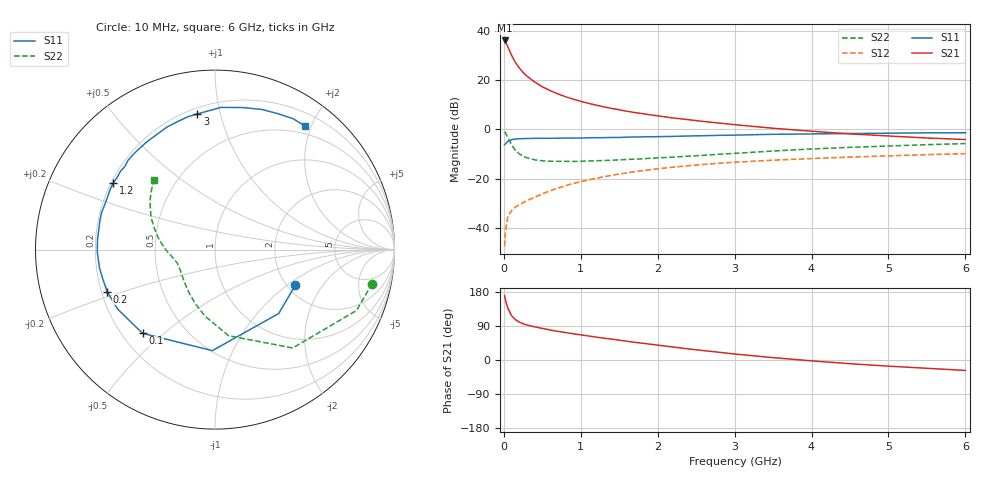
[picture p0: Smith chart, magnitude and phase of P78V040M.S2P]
! SIEMENS Small Signal Semiconductors
! BFP196
! Si NPN RF Bipolar Junction Transistor in SOT143
! VCE = 8 V  IC = 40 mA
! Common Emitter S-Parameters:  May  1996
# GHz  S  MA  R  50
!  f  S11  S21  S12  S22
! GHz  MAG  ANG  MAG  ANG  MAG  ANG  MAG  ANG
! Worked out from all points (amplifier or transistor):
!   36 points, 10 MHz to 6 GHz, reference 50 ohm
!   highest |S21| = 36.2 dB at 10 MHz (marker M1)
!   |S21| within 3 dB of that: start of sweep to 58.2 MHz
!   unconditionally stable (mu >= 1): 546.5 MHz to 4.494 GHz
!   at 250 MHz: K = 0.75, MSG = 26.5 dB, |S12| = -29.8 dB
!   at 1.4 GHz: K = 1.09, MAG = 11.8 dB, |S12| = -18.7 dB
!   at 6 GHz: K = 0.97, MSG = 2.9 dB, |S12| = -9.9 dB
!   S11 on the Smith chart (normalised r, x): 10 MHz: 2.22, -1.15; 100 MHz: 0.28, -0.43; 200 MHz: 0.22, -0.18; 1.2 GHz: 0.21, +0.29; 3 GHz: 0.24, +0.85; 6 GHz: 0.38, +1.91
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0.01  0.4898 -23.7  64.37 169.7  0.0042 79.7  0.8959 -12.2
0.02  0.5028 -45.1  60.9 159.5  0.0081 73.7  0.8581 -23.3
0.05  0.5632 -91.5  48.77 137.6  0.0164 57.4  0.6984 -51.7
0.1  0.6169 -130.9  32.24 117.0  0.0224 47.1  0.4859 -81.0
0.15  0.6358 -148.6  23.1 106.5  0.0263 45.9  0.3756 -98.4
0.2  0.6448 -158.7  17.86 100.1  0.0292 47.7  0.3186 -110.5
0.25  0.6467 -166.0  14.38 95.7  0.0322 48.8  0.283 -120.2
0.3  0.6514 -170.9  12.11 92.5  0.0354 50.9  0.2638 -127.0
0.4  0.6559 -178.8  9.188 87.5  0.0415 54.1  0.2405 -137.5
0.5  0.6571 175.3  7.354 83.3  0.0485 56.4  0.2293 -144.8
0.6  0.6567 170.5  6.146 79.3  0.0563 57.9  0.2248 -149.7
0.7  0.6615 165.5  5.289 75.5  0.0636 59.0  0.2235 -153.5
0.9  0.6631 157.8  4.116 69.4  0.0792 58.3  0.2225 -159.2
1.1  0.6732 150.4  3.384 63.4  0.0935 57.5  0.2272 -163.0
1.2  0.678 146.7  3.107 60.4  0.1011 56.7  0.2297 -164.7
1.7  0.6991 130.7  2.197 46.7  0.1374 51.0  0.2474 -172.5
2.2  0.7185 116.9  1.706 34.3  0.1699 44.3  0.2722 -179.3
3  0.7624 97.4  1.246 15.8  0.2147 32.9  0.325 167.7
3.5  0.793 87.6  1.053 6.2  0.2358 26.3  0.3621 159.9
4.5  0.8236 71.4  0.81 -9.8  0.2724 14.7  0.4302 147.0
5.5  0.8493 59.2  0.667 -21.9  0.3053 4.2  0.4878 136.4
6  0.8515 53.7  0.621 -27.6  0.3201 -1.5  0.5137 131.2
